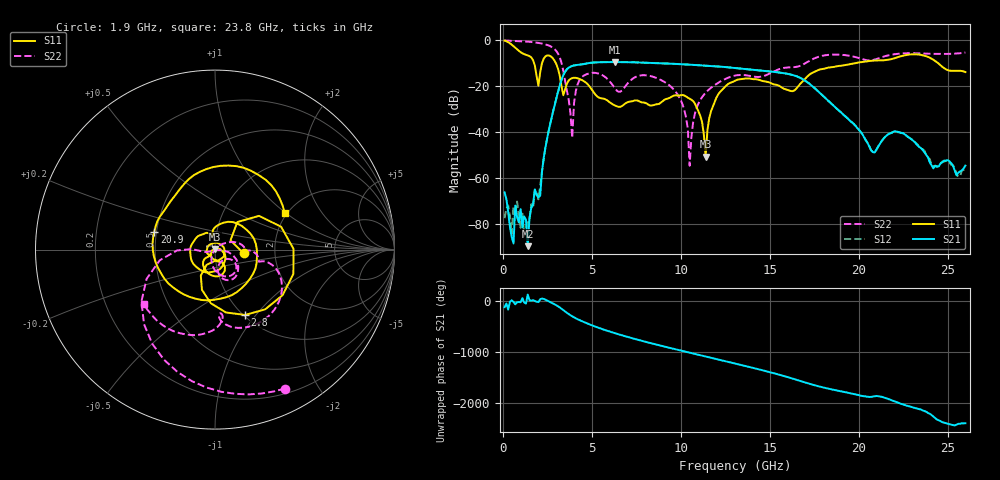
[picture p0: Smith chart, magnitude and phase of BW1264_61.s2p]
!Keysight Technologies,N5245B,MY57181159,A.13.60.06
!Date: Friday, December 18, 2020 23:55:15
!Correction: S11(Full 2 Port(1,2))
!S21(Full 2 Port(1,2))
!S12(Full 2 Port(1,2))
!S22(Full 2 Port(1,2))
!S2P File: Measurements: S11, S21, S12, S22:
# Hz S  dB  R 50
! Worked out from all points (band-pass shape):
!   260 points, 100 MHz to 26 GHz, reference 50 ohm
!   highest |S21| = -9.67 dB at 6.3 GHz (marker M1); lowest = -89.7 dB at 1.4 GHz (marker M2)
!   |S21| within 3 dB of the highest: 3.623 GHz to 13.53 GHz (9.904 GHz wide, 115 % of centre)
!   lowest |S11| = -50.8 dB at 11.4 GHz (marker M3), VSWR 1.01, Z = 50 + j0.289 ohm
!   |S11| at or under -10 dB: 1.747 GHz to 2.21 GHz (462.4 MHz wide, 23.4 % of centre); 2.969 GHz to 19.93 GHz (16.96 GHz wide, 148 % of centre); 24.44 GHz to end of sweep
!   |S22| runs from -54.7 to -0.3 dB; largest |S21 - S12| = 0.00075
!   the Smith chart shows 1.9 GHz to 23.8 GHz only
!   S11 on the Smith chart (normalised r, x): 1.9 GHz: 1.38, -0.06; 2.8 GHz: 1.02, -0.88; 20.9 GHz: 0.49, +0.11; 23.8 GHz: 1.94, +0.98
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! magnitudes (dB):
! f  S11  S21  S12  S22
! 100 MHz  -0.4  -66.3  -77.5  -0.3
! 400 MHz  -1.6  -81.4  -76.9  -0.4
! 1.4 GHz  -6.8  -89.7  -79.6  -0.8
! 1.9 GHz  -15.9  -67.4  -65.6  -1.2
! 2.8 GHz  -7.9  -31.9  -32.0  -3.4
! 3.4 GHz  -24.1  -15.3  -15.3  -13.5
! 3.9 GHz  -16.7  -11.4  -11.4  -42.6
! 4.1 GHz  -16.5  -11.0  -11.0  -22.4
! 4.5 GHz  -17.7  -10.6  -10.6  -15.8
! 6.3 GHz  -28.6  -9.7  -9.7  -21.1
! 8.8 GHz  -27.8  -10.2  -10.2  -17.2
! 10.1 GHz  -24.0  -10.6  -10.6  -28.1
! 10.5 GHz  -25.6  -10.8  -10.8  -54.7
! 10.8 GHz  -27.8  -11.0  -11.0  -32.0
! 11.4 GHz  -50.8  -11.2  -11.2  -23.0
! 11.9 GHz  -27.1  -11.5  -11.5  -19.7
! 13.1 GHz  -17.6  -12.3  -12.3  -15.5
! 17.4 GHz  -14.4  -20.2  -20.2  -8.5
! 20.9 GHz  -9.1  -49.0  -48.8  -8.6
! 21.7 GHz  -8.6  -40.9  -40.8  -6.7
! 23.8 GHz  -7.2  -50.1  -50.2  -6.0
! 26 GHz  -14.0  -54.7  -56.3  -5.6
